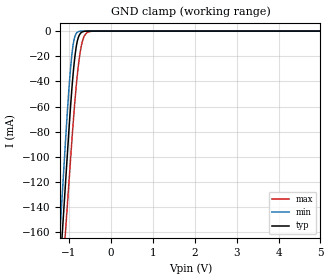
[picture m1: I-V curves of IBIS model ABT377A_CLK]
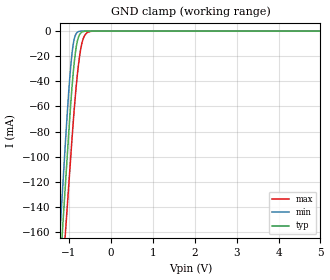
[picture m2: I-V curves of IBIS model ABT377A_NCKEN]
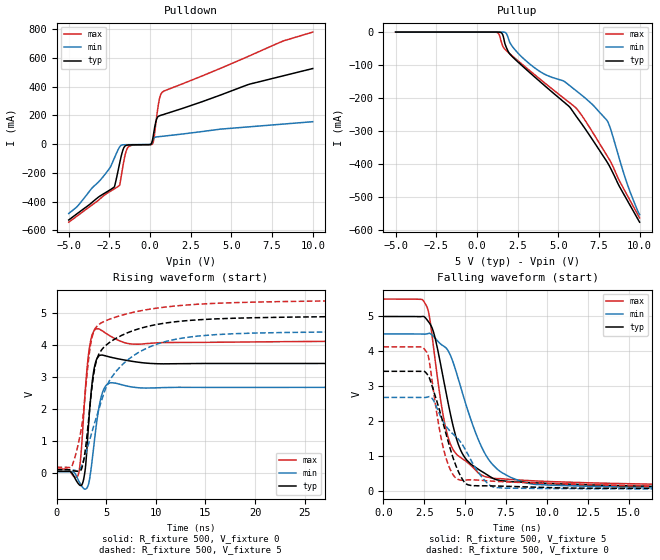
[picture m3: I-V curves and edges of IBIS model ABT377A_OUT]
| TEXAS INSTRUMENTS INCORPORATED
| Standard Linear and Logic Group
| IBIS Model of SN74ABT377A
| OCTAL EDGE-TRIGGERED D-TYPE FLIP-FLOPS WITH CLOCK ENABLE
| This file contains package information for the following:
|  SSOP 20-pin (DB) package as [Component] ABT377A_DB
|  SOIC 20-pin (DW) package as [Component] ABT377A_DW
|  PDIP 20-pin (N) package as [Component] ABT377A_N
|  TSSOP 20-pin (PW) package as [Component] ABT377A_PW
| This device can be powered at the following Vccs:
|  5 volt Vcc
| This file provides unique models under the [Model Selector] for each Vcc.
| For operation at a specific Vcc, select the appropriate model after each
| [Model Selector] keyword.
[IBIS Ver]   3.2
[Comment char]  |_char
[File Name]   sn74abt377a.ibs
[File Rev]   1.1 | n_die
[Date]   September 29, 2003
[Source]   Data created from TI-SPICE simulations at TI-SLL.
[Notes]   The following is an IBIS list for the ABT377A.
   Please contact sllibis@ti.com with questions and
   comments concerning SLL IBIS models.
   -This IBIS model is created from a BA (back annotated netlist)
   -Power clamp data deleted as there is no power-clamp diode.
   -C_comp values have been replaced by the data sheet typ values
   except for the output models.
   -We may not have accurate data for the weak case.
[Disclaimer] Property of Texas Instruments Incorporated.  Unauthorized
   reproduction and/or distribution is strictly prohibited.
   This product is protected under copyright law.
   Created  2002, (C) Copyright  2002, Texas Instruments
   Incorporated, All Rights Reserved
   UNLESS THERE IS A SIGNED, WRITTEN AGREEMENT TO THE
   CONTRARY, TEXAS INSTRUMENTS (TI) IS PROVIDING THE IBIS
   MODELS  AND WITHOUT ANY WARRANTY, EXPRESSED OR
   IMPLIED.  TI assumes no liability for:
   1) the accuracy of the IBIS models provided to your
   company;
   2) the proper functioning of these IBIS Models in your
   design or for any resulting applications; or
   3) infringement of patents, copyrights or intellectual
   property rights resulting from your use of these IBIS
   models.
   TI provides IBIS Models as a service to our customers.
   You and your company shall not distribute, sell or give
   these models to anyone else without prior written
   permission from TI.
   TI reserves the right to make changes to our products or
   to discontinue any semiconductor product or service
   without notice, and advises our customers to obtain the
   latest version of relevant information to verify, before
   placing orders, that the information being relied on is
   current.
   Please be aware that your receipt and use of the IBIS
   information provided shall serve as acceptance of these
   terms and conditions.  If you do not accept these terms,
   you should return or destroy the IBIS models and any
   other accompanying information immediately.
| Component ABT377A_DB 20-pin SSOP
[Component]   ABT377A_DB
[Manufacturer]   Texas Instruments, Inc.
[Package]
|   typ   min   max
R_pkg   4.000e-02   3.500e-02   5.100e-02
L_pkg   3.495e-09   3.035e-09   4.314e-09
C_pkg   4.200e-13   3.460e-13   5.020e-13
[Pin]   signal_name   model_name   R_pin   L_pin   C_pin
1   NCLKEN   ABT377A_NCKEN   4.900e-02   4.310e-09   5.020e-13
2   1Q   ABT377A_OUT   4.800e-02   3.903e-09   4.870e-13
3   1D   ABT377A_IN   3.500e-02   3.189e-09   3.960e-13
4   2D   ABT377A_IN   3.500e-02   3.036e-09   3.470e-13
5   2Q   ABT377A_OUT   3.500e-02   3.035e-09   3.670e-13
6   3Q   ABT377A_OUT   3.500e-02   3.035e-09   3.670e-13
7   3D   ABT377A_IN   3.500e-02   3.036e-09   3.470e-13
8   4D   ABT377A_IN   3.500e-02   3.189e-09   3.970e-13
9   4Q   ABT377A_OUT   4.700e-02   3.899e-09   4.880e-13
10   GND   GND   5.100e-02   4.314e-09   5.000e-13
11   CLK   ABT377A_CLK   5.100e-02   4.314e-09   5.000e-13
12   5Q   ABT377A_OUT   4.700e-02   3.899e-09   4.880e-13
13   5D   ABT377A_IN   3.500e-02   3.189e-09   3.970e-13
14   6D   ABT377A_IN   3.500e-02   3.036e-09   3.460e-13
15   6Q   ABT377A_OUT   3.500e-02   3.035e-09   3.670e-13
16   7Q   ABT377A_OUT   3.500e-02   3.035e-09   3.670e-13
17   7D   ABT377A_IN   3.500e-02   3.036e-09   3.460e-13
18   8D   ABT377A_IN   3.500e-02   3.189e-09   3.970e-13
19   8Q   ABT377A_OUT   4.700e-02   3.899e-09   4.880e-13
20   VCC   POWER   5.100e-02   4.314e-09   5.020e-13
| Component ABT377A_DW 20-pin SOIC
[Component]   ABT377A_DW
[Manufacturer]   Texas Instruments, Inc.
[Package]
|   typ   min   max
R_pkg   3.800e-02   3.300e-02   4.500e-02
L_pkg   5.012e-09   4.110e-09   6.349e-09
C_pkg   7.170e-13   5.300e-13   8.680e-13
[Pin]   signal_name   model_name   R_pin   L_pin   C_pin
1   NCLKEN   ABT377A_NCKEN   4.200e-02   6.336e-09   8.650e-13
2   1Q   ABT377A_OUT   4.300e-02   5.542e-09   8.670e-13
3   1D   ABT377A_IN   3.400e-02   4.714e-09   7.320e-13
4   2D   ABT377A_IN   3.400e-02   4.377e-09   5.910e-13
5   2Q   ABT377A_OUT   3.600e-02   4.130e-09   5.330e-13
6   3Q   ABT377A_OUT   3.500e-02   4.111e-09   5.300e-13
7   3D   ABT377A_IN   3.400e-02   4.284e-09   5.830e-13
8   4D   ABT377A_IN   3.400e-02   4.634e-09   7.260e-13
9   4Q   ABT377A_OUT   4.000e-02   5.518e-09   8.650e-13
10   GND   GND   4.300e-02   6.349e-09   8.660e-13
11   CLK   ABT377A_CLK   4.100e-02   6.281e-09   8.610e-13
12   5Q   ABT377A_OUT   4.500e-02   5.561e-09   8.680e-13
13   5D   ABT377A_IN   3.300e-02   4.778e-09   7.420e-13
14   6D   ABT377A_IN   3.500e-02   4.414e-09   5.960e-13
15   6Q   ABT377A_OUT   3.500e-02   4.110e-09   5.330e-13
16   7Q   ABT377A_OUT   3.600e-02   4.130e-09   5.330e-13
17   7D   ABT377A_IN   3.400e-02   4.377e-09   5.910e-13
18   8D   ABT377A_IN   3.400e-02   4.714e-09   7.310e-13
19   8Q   ABT377A_OUT   4.300e-02   5.569e-09   8.680e-13
20   VCC   POWER   4.200e-02   6.308e-09   8.640e-13
| Component ABT377A_N 20-pin PDIP
[Component]   ABT377A_N
[Manufacturer]   Texas Instruments, Inc.
[Package]
|   typ   min   max
R_pkg   4.300e-02   3.800e-02   5.000e-02
L_pkg   7.384e-09   4.680e-09   1.032e-08
C_pkg   5.100e-13   2.310e-13   8.210e-13
[Pin]   signal_name   model_name   R_pin   L_pin   C_pin
1   NCLKEN   ABT377A_NCKEN   4.200e-02   9.427e-09   8.100e-13
2   1Q   ABT377A_OUT   4.600e-02   8.544e-09   4.560e-13
3   1D   ABT377A_IN   4.800e-02   7.163e-09   4.350e-13
4   2D   ABT377A_IN   4.000e-02   4.825e-09   2.610e-13
5   2Q   ABT377A_OUT   4.000e-02   5.284e-09   6.480e-13
6   3Q   ABT377A_OUT   4.000e-02   4.686e-09   2.320e-13
7   3D   ABT377A_IN   4.000e-02   6.359e-09   4.890e-13
8   4D   ABT377A_IN   3.800e-02   7.982e-09   4.750e-13
9   4Q   ABT377A_OUT   4.300e-02   9.403e-09   4.750e-13
10   GND   GND   5.000e-02   1.032e-08   8.050e-13
11   CLK   ABT377A_CLK   5.000e-02   1.028e-08   8.100e-13
12   5Q   ABT377A_OUT   4.300e-02   9.383e-09   4.770e-13
13   5D   ABT377A_IN   3.800e-02   7.978e-09   4.760e-13
14   6D   ABT377A_IN   4.000e-02   6.302e-09   4.920e-13
15   6Q   ABT377A_OUT   4.000e-02   4.680e-09   2.310e-13
16   7Q   ABT377A_OUT   4.000e-02   5.284e-09   6.480e-13
17   7D   ABT377A_IN   4.000e-02   4.822e-09   2.610e-13
18   8D   ABT377A_IN   4.700e-02   7.118e-09   4.390e-13
19   8Q   ABT377A_OUT   4.600e-02   8.492e-09   4.610e-13
20   VCC   POWER   4.300e-02   9.348e-09   8.210e-13
| Component ABT377A_PW 20-pin TSSOP
[Component]   ABT377A_PW
[Manufacturer]   Texas Instruments, Inc.
[Package]
|   typ   min   max
R_pkg   5.000e-02   4.200e-02   6.000e-02
L_pkg   2.802e-09   2.248e-09   3.553e-09
C_pkg   3.170e-13   2.020e-13   4.430e-13
[Pin]   signal_name   model_name   R_pin   L_pin   C_pin
1   NCLKEN   ABT377A_NCKEN   5.500e-02   3.461e-09   4.400e-13
2   1Q   ABT377A_OUT   5.500e-02   3.150e-09   4.010e-13
3   1D   ABT377A_IN   4.200e-02   2.619e-09   3.020e-13
4   2D   ABT377A_IN   4.500e-02   2.273e-09   2.020e-13
5   2Q   ABT377A_OUT   4.500e-02   2.248e-09   2.240e-13
6   3Q   ABT377A_OUT   4.500e-02   2.273e-09   2.260e-13
7   3D   ABT377A_IN   4.400e-02   2.323e-09   2.050e-13
8   4D   ABT377A_IN   4.600e-02   2.704e-09   3.070e-13
9   4Q   ABT377A_OUT   6.000e-02   3.265e-09   4.110e-13
10   GND   GND   5.700e-02   3.506e-09   4.360e-13
11   CLK   ABT377A_CLK   5.800e-02   3.553e-09   4.370e-13
12   5Q   ABT377A_OUT   5.800e-02   3.193e-09   4.050e-13
13   5D   ABT377A_IN   4.200e-02   2.704e-09   3.110e-13
14   6D   ABT377A_IN   4.600e-02   2.392e-09   2.100e-13
15   6Q   ABT377A_OUT   4.700e-02   2.334e-09   2.290e-13
16   7Q   ABT377A_OUT   4.700e-02   2.300e-09   2.270e-13
17   7D   ABT377A_IN   4.700e-02   2.349e-09   2.070e-13
18   8D   ABT377A_IN   4.500e-02   2.677e-09   3.060e-13
19   8Q   ABT377A_OUT   6.000e-02   3.235e-09   4.060e-13
20   VCC   POWER   5.600e-02   3.487e-09   4.430e-13
| Models and submodels in the file (4): ABT377A_CLK (Input), ABT377A_IN (Input), ABT377A_NCKEN (Input), ABT377A_OUT (Output)
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[Model]   ABT377A_CLK
Model_type  Input
Vinl=0.8
Vinh=2.0
| variable   typ   min   max
C_comp   3.5pF   NA   NA
[Temperature Range]   40   -40   100
| Ambient temperature   25   -40   85
[Voltage range]   5   4.5   5.5
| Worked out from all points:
|   GND clamp passes 1 mA (typ) near -0.70 V on its own axis
[GND Clamp]
| ABT377A_CLK
|   Voltage   I(typ)   I(min)   I(max)
-5V       -2.153A    -2.252A    -2.029A
-1.27V    -219.8mA   -192.6mA   -250.3mA
-1.165V   -165.3mA   -134.6mA   -200.3mA
-1.075V   -118.7mA   -84.94mA   -157.4mA
-1V       -79.84mA   -47.06mA   -121.6mA
-925mV    -44.85mA   -17.94mA   -85.91mA
-850mV    -18.77mA   -3.745mA   -53.68mA
-775mV    -5.229mA   -456uA     -28.13mA
-725mV    -1.881mA   -65.53uA   -15.89mA
-650mV    -301.3uA   -1.883uA   -5.398mA
-475mV    -495.5nA   -657.9pA   -218.9uA
5V        60.29pA    64.86pA    153.2pA
[Model]   ABT377A_NCKEN
Model_type  Input
Vinl=0.8
Vinh=2.0
| variable   typ   min   max
C_comp   3.5pF   NA   NA
[Temperature Range]   40   -40   100
| Ambient temperature   25   -40   85
[Voltage range]   5   4.5   5.5
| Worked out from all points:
|   GND clamp passes 1 mA (typ) near -0.69 V on its own axis
[GND Clamp]
| ABT377A_NCKEN
|   Voltage   I(typ)   I(min)   I(max)
-5V       -2.154A    -2.253A    -2.03A
-1.275V   -222.5mA   -195.5mA   -252.9mA
-1.17V    -168mA     -137.5mA   -202.8mA
-1.075V   -118.8mA   -85mA      -157.5mA
-1V       -79.92mA   -47.11mA   -121.7mA
-925mV    -44.92mA   -17.98mA   -86mA
-850mV    -18.82mA   -3.769mA   -53.76mA
-775mV    -5.267mA   -468.9uA   -28.19mA
-725mV    -1.911mA   -71.29uA   -15.94mA
-650mV    -319.5uA   -2.351uA   -5.436mA
-475mV    -1.1uA     -759.2pA   -229.6uA
5V        213.6pA    214.9pA    332.4pA
[Model]   ABT377A_OUT
Model_type  Output
Vref =   0
Rref =   500
Cref =   50p
Vmeas =   1.5
| variable   typ   min   max
C_comp   11.61pF   1.41pF   52.34pF
| C_pullup   7.09pF   1.55pF   9.81pF
| C_pulldown   16.13pF   1.41pF   52.34pF
[Temperature Range]   40   -40   100
| Ambient temperature   25   -40   85
[Voltage range]   5   4.5   5.5
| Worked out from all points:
|   slope of the pulldown table from 0 to 0.75 V, typ, clamps not added: 3.63 ohm
|   rising waveform, R_fixture 500, V_fixture 0: 20-80 % time 508ps typ, 684ps min, 544ps max; typ from 0.056 V to 3.42 V
|   falling waveform, R_fixture 500, V_fixture 5: 20-80 % time 1.48ns typ, 2.01ns min, 1.21ns max; typ from 5 V to 0.107 V
|   rising waveform, R_fixture 500, V_fixture 5: 20-80 % time 1.87ns typ, 4.06ns min, 1.32ns max; typ from 0.106 V to 4.93 V
|   falling waveform, R_fixture 500, V_fixture 0: 20-80 % time 1.28ns typ, 2.27ns min, 910ps max; typ from 3.43 V to 0.058 V
[Pulldown]
| ABT377A_OUT
|   Voltage   I(typ)   I(min)   I(max)
-5V       -527.2mA   -481.9mA   -542.6mA
-2.91V    -348.7mA   -229.4mA   -363.6mA
-2.195V   -296.8mA   -96.54mA   -310.7mA
-1.875V   -135.1mA   -19.79mA   -285.6mA
-1.8V     -96.32mA   -9.545mA   -241.8mA
-1.54V    -12.91mA   -3.633mA   -77.55mA
-1.345V   -5.687mA   -3.229mA   -20.09mA
145mV     26.66mA    22.15mA    2.066mA
425mV     181.3mA    51.07mA    208.9mA
580mV     197.8mA    53mA       317.6mA
750mV     204.2mA    55.05mA    362mA
10V       526.6mA    156.7mA    780.2mA
[Pullup]
| ABT377A_OUT
|   Voltage   I(typ)   I(min)   I(max)
-5V       1.608uA    1.522nA    35.81uA
1.18V     -6.091uA   -574.2pA   -500.3uA
1.36V     -167.9uA   -104.2nA   -7.156mA
1.545V    -4.41mA    -9.98uA    -36.58mA
1.76V     -40.59mA   -1.68mA    -53.86mA
2.22V     -76.56mA   -46.35mA   -74.12mA
3.23V     -121.8mA   -95.93mA   -116mA
5.65V     -224.2mA   -159.8mA   -211.8mA
6.09V     -253.6mA   -177mA     -229.6mA
7.99V     -392.1mA   -267mA     -373.3mA
9.255V    -510.2mA   -461.8mA   -495mA
10V       -575mA     -552.2mA   -562.2mA
[Ramp]
| ABT377A_OUT
| variable   typ   min   max
dV/dt_r   2.44/6.42E-10   1.99/8.60E-10   2.78/6.62E-10
dV/dt_f   2.94/1.49E-09   2.65/2.04E-09   3.20/1.24E-09
R_load = 500
[Rising Waveform]
| ABT377A_OUT
R_fixture =   500
C_fixture =   0
L_fixture =   0
V_fixture =   0
V_fixture_min = 0
V_fixture_max = 0
|   Time   V(typ)   V(min)   V(max)
0s        56.14mV    43.81mV    126mV
2.115ns   -296mV     -165.6mV   -103.6mV
2.625ns   -318.6mV   -444.1mV   1.286V
2.915ns   180.5mV    -501.2mV   2.661V
3.25ns    1.608V     -315.4mV   3.771V
3.6ns     2.854V     431.3mV    4.325V
3.97ns    3.493V     1.405V     4.503V
4.625ns   3.684V     2.51V      4.438V
5.49ns    3.615V     2.822V     4.265V
50ns      3.425V     2.677V     4.126V
[Falling Waveform]
| ABT377A_OUT
R_fixture =   500
C_fixture =   0
L_fixture =   0
V_fixture =   5
V_fixture_min = 4.5
V_fixture_max = 5.5
|   Time   V(typ)   V(min)   V(max)
0s        5V         4.5V       5.5V
2.525ns   4.984V     4.494V     5.394V
2.79ns    4.829V     4.519V     5.061V
3.105ns   4.486V     4.409V     3.973V
3.61ns    3.36V      4.173V     2.287V
4.045ns   2.324V     3.941V     1.41V
4.845ns   1.054V     2.79V      911.5mV
6.32ns    465.4mV    979.9mV    393.2mV
10.25ns   207.1mV    158.6mV    262.2mV
50ns      107mV      97.24mV    181.4mV
[Rising Waveform]
| ABT377A_OUT
R_fixture =   500
C_fixture =   0
L_fixture =   0
V_fixture =   5
V_fixture_min = 4.5
V_fixture_max = 5.5
|   Time   V(typ)   V(min)   V(max)
0s        106.1mV    96.66mV    181.1mV
1.525ns   91.83mV    97.62mV    198.8mV
2.5ns     110.8mV    206.6mV    1.39V
2.925ns   787.8mV    591mV      2.593V
3.645ns   2.865V     1.365V     4.315V
4.28ns    3.723V     2.009V     4.645V
5.835ns   4.178V     3.11V      4.858V
9.215ns   4.582V     3.917V     5.109V
14.44ns   4.789V     4.284V     5.276V
50ns      4.931V     4.441V     5.433V
[Falling Waveform]
| ABT377A_OUT
R_fixture =   500
C_fixture =   0
L_fixture =   0
V_fixture =   0
V_fixture_min = 0
V_fixture_max = 0
|   Time   V(typ)   V(min)   V(max)
0s        3.427V     2.678V     4.129V
2.665ns   3.351V     2.683V     3.968V
3.05ns    2.897V     2.606V     2.913V
3.73ns    1.809V     1.925V     1.105V
4.21ns    1.02V      1.649V     500mV
4.72ns    423mV      1.397V     304.3mV
5.16ns    172.7mV    1.051V     311.6mV
6.245ns   141.2mV    271.2mV    288.2mV
7.335ns   130mV      75.27mV    257.9mV
50ns      57.86mV    45.2mV     126.9mV
